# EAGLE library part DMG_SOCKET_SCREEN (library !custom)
DMG Flex Cable Connecter This part does not have any spec that can be found. Part was measured with a caliper with a resolution of .5mil. Pad spacing is at 50mil.
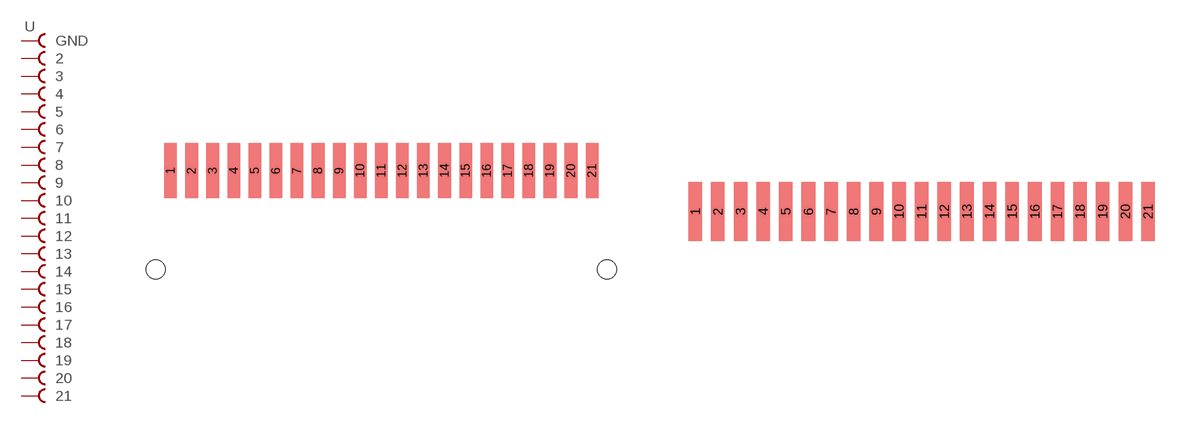
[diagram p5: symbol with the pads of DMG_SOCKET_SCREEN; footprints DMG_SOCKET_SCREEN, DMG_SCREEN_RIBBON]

Designator prefix -

## DMG_SOCKET_SCREEN  [DMG_SOCKET_SCREEN]
1  GND  pas
2  2  pas
3  3  pas
4  4  pas
5  5  pas
6  6  pas
7  7  pas
8  8  pas
9  9  pas
10  10  pas
11  11  pas
12  12  pas
13  13  pas
14  14  pas
15  15  pas
16  16  pas
17  17  pas
18  18  pas
19  19  pas
20  20  pas
21  21  pas

## DMG_SOCKET_SCREEN_RIBBON  [DMG_SCREEN_RIBBON]
Pads as for DMG_SOCKET_SCREEN

## Footprint DMG_SOCKET_SCREEN (pad centres in mm)
smd 0.762 x 3.302: 1 -12.7,5.969; 2 -11.43,5.969; 3 -10.16,5.969; 4 -8.89,5.969; 5 -7.62,5.969; 6 -6.35,5.969; 7 -5.08,5.969; 8 -3.81,5.969; 9 -2.54,5.969; 10 -1.27,5.969; 11 0,5.969; 12 1.27,5.969; 13 2.54,5.969; 14 3.81,5.969; 15 5.08,5.969; 16 6.35,5.969; 17 7.62,5.969; 18 8.89,5.969; 19 10.16,5.969; 20 11.43,5.969; 21 12.7,5.969
hole 1.143 at -13.589,0
hole 1.143 at 13.589,0

## Footprint DMG_SCREEN_RIBBON (pad centres in mm)
smd 0.762 x 3.302: 1 -12.7,0; 2 -11.43,0; 3 -10.16,0; 4 -8.89,0; 5 -7.62,0; 6 -6.35,0; 7 -5.08,0; 8 -3.81,0; 9 -2.54,0; 10 -1.27,0; 11 0,0; 12 1.27,0; 13 2.54,0; 14 3.81,0; 15 5.08,0; 16 6.35,0; 17 7.62,0; 18 8.89,0; 19 10.16,0; 20 11.43,0; 21 12.7,0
